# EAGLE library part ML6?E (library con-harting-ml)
HARTING
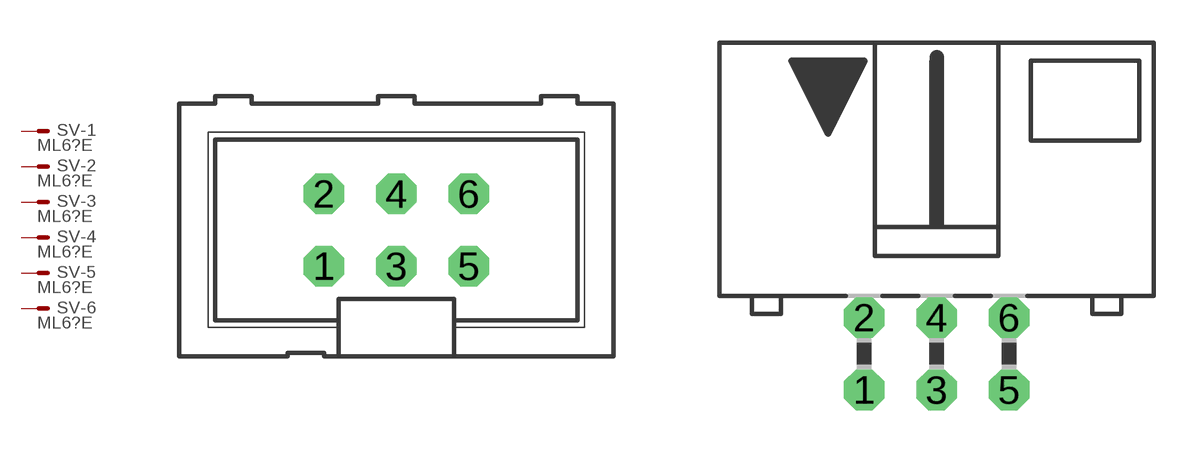
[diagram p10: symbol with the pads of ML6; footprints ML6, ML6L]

Designator prefix SV; gates -1=M -2=M -3=M -4=M -5=M -6=M

## ML6E (OC_FARNELL: unknown; OC_NEWARK: unknown)  [ML6]
1  -1:S  pas
2  -2:S  pas
3  -3:S  pas
4  -4:S  pas
5  -5:S  pas
6  -6:S  pas

## ML6LE (OC_FARNELL: unknown; OC_NEWARK: unknown)  [ML6L]
Pads as for ML6

## Footprint ML6 (pad centres in mm)
HARTING
drill 0.914 octagon: 1 -2.54,-1.27; 2 -2.54,1.27; 3 0,-1.27; 4 0,1.27; 5 2.54,-1.27; 6 2.54,1.27

## Footprint ML6L (pad centres in mm)
HARTING
drill 0.914 octagon: 1 -2.54,-1.27; 2 -2.54,1.27; 3 0,-1.27; 4 0,1.27; 5 2.54,-1.27; 6 2.54,1.27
